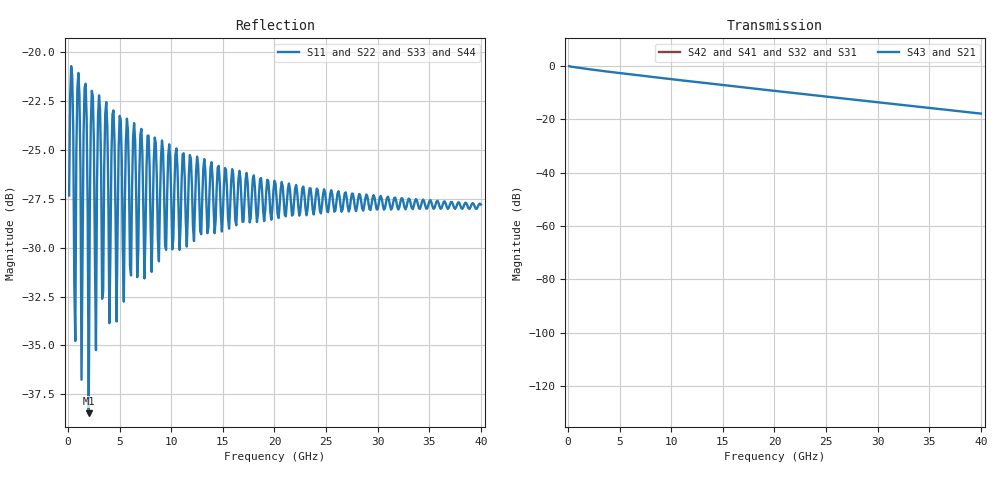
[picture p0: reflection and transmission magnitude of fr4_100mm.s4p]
! Touchstone Ver. 1.0
! Number of ports is 4
! port1 ->  port2
! port3 ->  port4
# Hz	S	RI	R	50.000000
! SCATTERING PARAMETERS  :
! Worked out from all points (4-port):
!   400 points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, 100 MHz to 40 GHz, reference 50 ohm
!   strongest paths, dB at 100 MHz, 10.1 GHz, 20.1 GHz, 30.1 GHz, 40 GHz:
!     S43: -0.2, -5.1, -9.4, -13.7, -17.9
!     S21: -0.2, -5.1, -9.4, -13.7, -17.9
!     S42: -, -, -, -, -
!     S41: -, -, -, -, -
!     S32: -, -, -, -, -
!     S31: -, -, -, -, -
!   lowest |S11| = -38.5 dB at 2 GHz (marker M1), VSWR 1.02, Z = 48.8 + j0.074 ohm
!   |S11| at or under -10 dB: start of sweep to end of sweep
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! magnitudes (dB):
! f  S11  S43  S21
! 100 MHz  -27.3  -0.2  -0.2
! 1 GHz  -21.1  -0.8  -0.8
! 1.3 GHz  -36.8  -0.9  -0.9
! 1.7 GHz  -21.6  -1.1  -1.1
! 2 GHz  -38.5  -1.3  -1.3
! 2.3 GHz  -22.0  -1.4  -1.4
! 40 GHz  -27.8  -17.9  -17.9
